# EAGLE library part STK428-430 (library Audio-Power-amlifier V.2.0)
SANYO CLASS-D AUDIO 2x150W POWER AMPLIFIERS
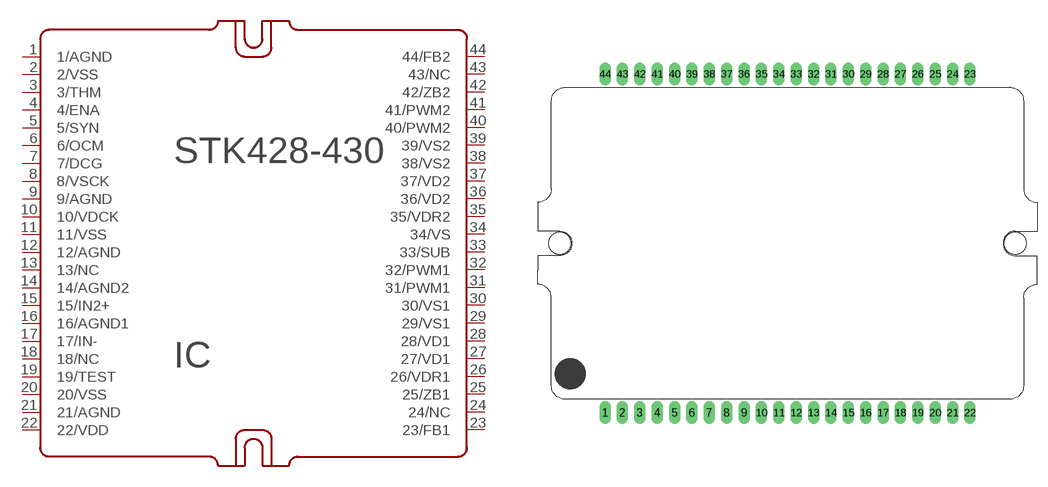
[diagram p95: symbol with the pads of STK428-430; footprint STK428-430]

Designator prefix IC

## STK428-430  [STK428-430]
1  1/AGND  pwr
2  2/VSS  pwr
3  3/THM
4  4/ENA
5  5/SYN
6  6/OCM
7  7/DCG
8  8/VSCK
9  9/AGND  pwr
10  10/VDCK
11  11/VSS  pwr
12  12/AGND  pwr
13  13/NC  nc
14  14/AGND2  pwr
15  15/IN2+  in
16  16/AGND1  pwr
17  17/IN-  in
18  18/NC  nc
19  19/TEST
20  20/VSS  pwr
21  21/AGND  pwr
22  22/VDD  pwr
23  23/FB1
24  24/NC  nc
25  25/ZB1
26  26/VDR1
27  27/VD1
28  28/VD1
29  29/VS1
30  30/VS1
31  31/PWM1
32  32/PWM1
33  33/SUB
34  34/VS
35  35/VDR2
36  36/VD2
37  37/VD2
38  38/VS2
39  39/VS2
40  40/PWM2
41  41/PWM2
42  42/ZB2
43  43/NC  nc
44  44/FB2

## Footprint STK428-430 (pad centres in mm)
drill 0.7 pad 1.676 long: 1 -26.67,-24.75; 2 -24.13,-24.75; 3 -21.59,-24.75; 4 -19.05,-24.75; 5 -16.51,-24.75; 6 -13.97,-24.75; 7 -11.43,-24.75; 8 -8.89,-24.75; 9 -6.35,-24.75; 10 -3.81,-24.75; 11 -1.27,-24.75; 12 1.27,-24.75; 13 3.81,-24.75; 14 6.35,-24.75; 15 8.89,-24.75; 16 11.43,-24.75; 17 13.97,-24.75; 18 16.51,-24.75; 19 19.05,-24.75; 20 21.59,-24.75; 21 24.13,-24.75; 22 26.67,-24.75; 23 26.67,24.75; 24 24.13,24.75; 25 21.59,24.75; 26 19.05,24.75; 27 16.51,24.75; 28 13.97,24.75; 29 11.43,24.75; 30 8.89,24.75; 31 6.35,24.75; 32 3.81,24.75; 33 1.27,24.75; 34 -1.27,24.75; 35 -3.81,24.75; 36 -6.35,24.75; 37 -8.89,24.75; 38 -11.43,24.75; 39 -13.97,24.75; 40 -16.51,24.75; 41 -19.05,24.75; 42 -21.59,24.75; 43 -24.13,24.75; 44 -26.67,24.75
hole 3.2 at -33.28,0
hole 3.2 at 33.29,-0.01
